| IBIS file stm32u575_585_lqfp64.ibs
[IBIS ver] 4.2
[File name] stm32u575_585_lqfp64.ibs
[File Rev] 1.0
[Date]   06-08-2021
[Source] Data Created at STMicroelectronics
[Notes]  File originated from ELDO simulations.
[Disclaimer]  This information is for modeling purpose only and is
   not guaranted. The information is subject to change without
   notice.
[Copyright] Copyright 2021 STMicroelectronics Inc.
|   Component stm32u575_585_lqfp64
[Component] stm32u575_585_lqfp64
[Manufacturer] STMicroelectronics
[Package]
| variable   typ   min   max
R_pkg   0   NA   NA
L_pkg   0   NA   NA
C_pkg   0   NA   NA
[Pin]   signal_name   model_name   R_pin   L_pin   C_pin   | Comment
1 VBAT POWER 68.980E-3 4.220E-9 120.000E-15
2 PC13 io8_100m_ft_v33 63.756E-3 3.679E-9 93.469E-15
3 PC14-OSC32_IN io8_100m_ft 59.336E-3 3.221E-9 71.020E-15
4 PC15-OSC32_OUT io8_100m_ft 55.719E-3 2.846E-9 52.653E-15
5 PH0-OSC_IN io8_100m_ft 52.907E-3 2.555E-9 38.367E-15
6 PH1-OSC_OUT io8_100m_ft 50.897E-3 2.347E-9 28.163E-15
7 NRST nc 49.692E-3 2.222E-9 22.041E-15
8 PC0 io8_100m_hslv_ft 49.290E-3 2.180E-9 20.000E-15
9 PC1 io8_166m_hslv_i2c_ft 49.290E-3 2.180E-9 20.000E-15
10 PC2 io8_100m_hslv_ft 49.692E-3 2.222E-9 22.041E-15
11 PC3 io8_100m_hslv_ft 50.897E-3 2.347E-9 28.163E-15
12 VSSA GND 52.907E-3 2.555E-9 38.367E-15
13 VDDA POWER 55.719E-3 2.846E-9 52.653E-15
14 PA0 io8_100m_hslv_tamp_ft 59.336E-3 3.221E-9 71.020E-15
15 PA1 io8_100m_hslv_tamp_ft 63.756E-3 3.679E-9 93.469E-15
16 PA2 io8_100m_hslv_ft 68.980E-3 4.220E-9 120.000E-15
17 PA3 io8_166m_hslv_ft 68.980E-3 4.220E-9 120.000E-15
18 VSS GND 63.756E-3 3.679E-9 93.469E-15
19 VDD POWER 59.336E-3 3.221E-9 71.020E-15
20 PA4 io8_100m_hslv_ft 55.719E-3 2.846E-9 52.653E-15
21 PA5 io8_100m_ft 52.907E-3 2.555E-9 38.367E-15
22 PA6 io8_100m_hslv_ft 50.897E-3 2.347E-9 28.163E-15
23 PA7 io8_100m_hslv_ft 49.692E-3 2.222E-9 22.041E-15
24 PC4 io8_100m_hslv_ft 49.290E-3 2.180E-9 20.000E-15
25 PC5 io8_100m_tamp_ft 49.290E-3 2.180E-9 20.000E-15
26 PB0 io8_100m_hslv_ft 49.692E-3 2.222E-9 22.041E-15
27 PB1 io8_100m_hslv_ft 50.897E-3 2.347E-9 28.163E-15
28 PB2 io8_100m_hslv_tamp_ft 52.907E-3 2.555E-9 38.367E-15
29 PB10 io8_166m_hslv_i2c_ft 55.719E-3 2.846E-9 52.653E-15
30 VCAP POWER 59.336E-3 3.221E-9 71.020E-15
31 VSS GND 63.756E-3 3.679E-9 93.469E-15
32 VDD POWER 68.980E-3 4.220E-9 120.000E-15
33 PB12 io8_166m_hslv_ft 68.980E-3 4.220E-9 120.000E-15
34 PB13 io8_100m_i2c_ft 63.756E-3 3.679E-9 93.469E-15
35 PB14 io8_100m_i2c_ft 59.336E-3 3.221E-9 71.020E-15
36 PB15 nc 55.719E-3 2.846E-9 52.653E-15
37 PC6 io8_100m_ft 52.907E-3 2.555E-9 38.367E-15
38 PC7 io8_100m_ft 50.897E-3 2.347E-9 28.163E-15
39 PC8 io8_100m_ft 49.692E-3 2.222E-9 22.041E-15
40 PC9 io8_100m_ft 49.290E-3 2.180E-9 20.000E-15
41 PA8 io8_166m_hslv_ft 49.290E-3 2.180E-9 20.000E-15
42 PA9 io8_100m_usb_vbus_ft 49.692E-3 2.222E-9 22.041E-15
43 PA10 io8_100m_usb_id 50.897E-3 2.347E-9 28.163E-15
44 PA11 io8_usb_ft 52.907E-3 2.555E-9 38.367E-15
45 PA12 io8_usb_ft 55.719E-3 2.846E-9 52.653E-15
46 PA13 io8_100m_ft 59.336E-3 3.221E-9 71.020E-15
47 VSSUSB GND 63.756E-3 3.679E-9 93.469E-15
48 VDDUSB POWER 68.980E-3 4.220E-9 120.000E-15
49 PA14 io8_100m_ft 68.980E-3 4.220E-9 120.000E-15
50 PA15 nc 63.756E-3 3.679E-9 93.469E-15
51 PC10 io8_100m_ft 59.336E-3 3.221E-9 71.020E-15
52 PC11 io8_100m_hslv_ft 55.719E-3 2.846E-9 52.653E-15
53 PC12 io8_166m_hslv_ft 52.907E-3 2.555E-9 38.367E-15
54 PD2 io8_100m_ft 50.897E-3 2.347E-9 28.163E-15
55 PB3 io8_100m_i2c_ft 49.692E-3 2.222E-9 22.041E-15
56 PB4 io8_100m_i2c_ft 49.290E-3 2.180E-9 20.000E-15
57 PB5 io8_166m_hslv_ft 49.290E-3 2.180E-9 20.000E-15
58 PB6 io8_100m_i2c_ft 49.692E-3 2.222E-9 22.041E-15
59 PB7 io8_166m_hslv_i2c_ft 50.897E-3 2.347E-9 28.163E-15
60 PH3-BOOT0 io8_100m_ft 52.907E-3 2.555E-9 38.367E-15
61 PB8 io8_100m_i2c_ft 55.719E-3 2.846E-9 52.653E-15
62 PB9 io8_100m_i2c_ft 59.336E-3 3.221E-9 71.020E-15
63 VSS GND 63.756E-3 3.679E-9 93.469E-15
64 VDD POWER 68.980E-3 4.220E-9 120.000E-15
[Model Selector] io8_100m_ft
io8_100m_ft_hs_1v2  "IO8_FT 100MHz high speed @ 1.2V"
io8_100m_ft_hs_pu_1v2  "IO8_FT 100MHz high speed @ 1.2V pullup"
io8_100m_ft_hs_pd_1v2  "IO8_FT 100MHz high speed @ 1.2V pulldown"
io8_100m_ft_fs_1v2  "IO8_FT 100MHz fast speed @ 1.2V"
io8_100m_ft_fs_pu_1v2  "IO8_FT 100MHz fast speed @ 1.2V pullup"
io8_100m_ft_fs_pd_1v2  "IO8_FT 100MHz fast speed @ 1.2V pulldown"
io8_100m_ft_ms_1v2  "IO8_FT 100MHz med speed @ 1.2V"
io8_100m_ft_ms_pu_1v2  "IO8_FT 100MHz med speed @ 1.2V pullup"
io8_100m_ft_ms_pd_1v2  "IO8_FT 100MHz med speed @ 1.2V pulldown"
io8_100m_ft_ls_1v2  "IO8_FT 100MHz low speed @ 1.2V"
io8_100m_ft_ls_pu_1v2  "IO8_FT 100MHz low speed @ 1.2V pullup"
io8_100m_ft_ls_pd_1v2  "IO8_FT 100MHz low speed @ 1.2V pulldown"
io8_100m_ft_hs_1v8  "IO8_FT 100MHz high speed @ 1.8V"
io8_100m_ft_hs_pu_1v8  "IO8_FT 100MHz high speed @ 1.8V pullup"
io8_100m_ft_hs_pd_1v8  "IO8_FT 100MHz high speed @ 1.8V pulldown"
io8_100m_ft_fs_1v8  "IO8_FT 100MHz fast speed @ 1.8V"
io8_100m_ft_fs_pu_1v8  "IO8_FT 100MHz fast speed @ 1.8V pullup"
io8_100m_ft_fs_pd_1v8  "IO8_FT 100MHz fast speed @ 1.8V pulldown"
io8_100m_ft_ms_1v8  "IO8_FT 100MHz med speed @ 1.8V"
io8_100m_ft_ms_pu_1v8  "IO8_FT 100MHz med speed @ 1.8V pullup"
io8_100m_ft_ms_pd_1v8  "IO8_FT 100MHz med speed @ 1.8V pulldown"
io8_100m_ft_ls_1v8  "IO8_FT 100MHz low speed @ 1.8V"
io8_100m_ft_ls_pu_1v8  "IO8_FT 100MHz low speed @ 1.8V pullup"
io8_100m_ft_ls_pd_1v8  "IO8_FT 100MHz low speed @ 1.8V pulldown"
io8_100m_ft_hs_3v3  "IO8_FT 100MHz high speed @ 3.3V"
io8_100m_ft_hs_pu_3v3  "IO8_FT 100MHz high speed @ 3.3V pullup"
io8_100m_ft_hs_pd_3v3  "IO8_FT 100MHz high speed @ 3.3V pulldown"
io8_100m_ft_fs_3v3  "IO8_FT 100MHz fast speed @ 3.3V"
io8_100m_ft_fs_pu_3v3  "IO8_FT 100MHz fast speed @ 3.3V pullup"
io8_100m_ft_fs_pd_3v3  "IO8_FT 100MHz fast speed @ 3.3V pulldown"
io8_100m_ft_ms_3v3  "IO8_FT 100MHz med speed @ 3.3V"
io8_100m_ft_ms_pu_3v3  "IO8_FT 100MHz med speed @ 3.3V pullup"
io8_100m_ft_ms_pd_3v3  "IO8_FT 100MHz med speed @ 3.3V pulldown"
io8_100m_ft_ls_3v3  "IO8_FT 100MHz low speed @ 3.3V"
io8_100m_ft_ls_pu_3v3  "IO8_FT 100MHz low speed @ 3.3V pullup"
io8_100m_ft_ls_pd_3v3  "IO8_FT 100MHz low speed @ 3.3V pulldown"
[Model Selector] io8_100m_hslv_ft
io8_100m_ft_hs_1v2  "IO8_FT 100MHz high speed @ 1.2V"
io8_100m_ft_hs_pu_1v2  "IO8_FT 100MHz high speed @ 1.2V pullup"
io8_100m_ft_hs_pd_1v2  "IO8_FT 100MHz high speed @ 1.2V pulldown"
io8_100m_ft_fs_1v2  "IO8_FT 100MHz fast speed @ 1.2V"
io8_100m_ft_fs_pu_1v2  "IO8_FT 100MHz fast speed @ 1.2V pullup"
io8_100m_ft_fs_pd_1v2  "IO8_FT 100MHz fast speed @ 1.2V pulldown"
io8_100m_ft_ms_1v2  "IO8_FT 100MHz med speed @ 1.2V"
io8_100m_ft_ms_pu_1v2  "IO8_FT 100MHz med speed @ 1.2V pullup"
io8_100m_ft_ms_pd_1v2  "IO8_FT 100MHz med speed @ 1.2V pulldown"
io8_100m_ft_ls_1v2  "IO8_FT 100MHz low speed @ 1.2V"
io8_100m_ft_ls_pu_1v2  "IO8_FT 100MHz low speed @ 1.2V pullup"
io8_100m_ft_ls_pd_1v2  "IO8_FT 100MHz low speed @ 1.2V pulldown"
io8_100m_ft_hs_1v8  "IO8_FT 100MHz high speed @ 1.8V"
io8_100m_ft_hs_pu_1v8  "IO8_FT 100MHz high speed @ 1.8V pullup"
io8_100m_ft_hs_pd_1v8  "IO8_FT 100MHz high speed @ 1.8V pulldown"
io8_100m_ft_fs_1v8  "IO8_FT 100MHz fast speed @ 1.8V"
io8_100m_ft_fs_pu_1v8  "IO8_FT 100MHz fast speed @ 1.8V pullup"
io8_100m_ft_fs_pd_1v8  "IO8_FT 100MHz fast speed @ 1.8V pulldown"
io8_100m_ft_ms_1v8  "IO8_FT 100MHz med speed @ 1.8V"
io8_100m_ft_ms_pu_1v8  "IO8_FT 100MHz med speed @ 1.8V pullup"
io8_100m_ft_ms_pd_1v8  "IO8_FT 100MHz med speed @ 1.8V pulldown"
io8_100m_ft_ls_1v8  "IO8_FT 100MHz low speed @ 1.8V"
io8_100m_ft_ls_pu_1v8  "IO8_FT 100MHz low speed @ 1.8V pullup"
io8_100m_ft_ls_pd_1v8  "IO8_FT 100MHz low speed @ 1.8V pulldown"
io8_100m_ft_hs_3v3  "IO8_FT 100MHz high speed @ 3.3V"
io8_100m_ft_hs_pu_3v3  "IO8_FT 100MHz high speed @ 3.3V pullup"
io8_100m_ft_hs_pd_3v3  "IO8_FT 100MHz high speed @ 3.3V pulldown"
io8_100m_ft_fs_3v3  "IO8_FT 100MHz fast speed @ 3.3V"
io8_100m_ft_fs_pu_3v3  "IO8_FT 100MHz fast speed @ 3.3V pullup"
io8_100m_ft_fs_pd_3v3  "IO8_FT 100MHz fast speed @ 3.3V pulldown"
io8_100m_ft_ms_3v3  "IO8_FT 100MHz med speed @ 3.3V"
io8_100m_ft_ms_pu_3v3  "IO8_FT 100MHz med speed @ 3.3V pullup"
io8_100m_ft_ms_pd_3v3  "IO8_FT 100MHz med speed @ 3.3V pulldown"
io8_100m_ft_ls_3v3  "IO8_FT 100MHz low speed @ 3.3V"
io8_100m_ft_ls_pu_3v3  "IO8_FT 100MHz low speed @ 3.3V pullup"
io8_100m_ft_ls_pd_3v3  "IO8_FT 100MHz low speed @ 3.3V pulldown"
io8_100m_hslv_ft_hs_1v2  "IO8_FT 100MHz HSLV high speed @ 1.2V"
io8_100m_hslv_ft_hs_pu_1v2  "IO8_FT 100MHz HSLV high speed @ 1.2V pullup"
io8_100m_hslv_ft_hs_pd_1v2  "IO8_FT 100MHz HSLV high speed @ 1.2V pulldown"
io8_100m_hslv_ft_fs_1v2  "IO8_FT 100MHz HSLV fast speed @ 1.2V"
io8_100m_hslv_ft_fs_pu_1v2  "IO8_FT 100MHz HSLV fast speed @ 1.2V pullup"
io8_100m_hslv_ft_fs_pd_1v2  "IO8_FT 100MHz HSLV fast speed @ 1.2V pulldown"
io8_100m_hslv_ft_ms_1v2  "IO8_FT 100MHz HSLV med speed @ 1.2V"
io8_100m_hslv_ft_ms_pu_1v2  "IO8_FT 100MHz HSLV med speed @ 1.2V pullup"
io8_100m_hslv_ft_ms_pd_1v2  "IO8_FT 100MHz HSLV med speed @ 1.2V pulldown"
io8_100m_hslv_ft_ls_1v2  "IO8_FT 100MHz HSLV low speed @ 1.2V"
io8_100m_hslv_ft_ls_pu_1v2  "IO8_FT 100MHz HSLV low speed @ 1.2V pullup"
io8_100m_hslv_ft_ls_pd_1v2  "IO8_FT 100MHz HSLV low speed @ 1.2V pulldown"
io8_100m_hslv_ft_hs_1v8  "IO8_FT 100MHz HSLV high speed @ 1.8V"
io8_100m_hslv_ft_hs_pu_1v8  "IO8_FT 100MHz HSLV high speed @ 1.8V pullup"
io8_100m_hslv_ft_hs_pd_1v8  "IO8_FT 100MHz HSLV high speed @ 1.8V pulldown"
io8_100m_hslv_ft_fs_1v8  "IO8_FT 100MHz HSLV fast speed @ 1.8V"
io8_100m_hslv_ft_fs_pu_1v8  "IO8_FT 100MHz HSLV fast speed @ 1.8V pullup"
io8_100m_hslv_ft_fs_pd_1v8  "IO8_FT 100MHz HSLV fast speed @ 1.8V pulldown"
io8_100m_hslv_ft_ms_1v8  "IO8_FT 100MHz HSLV med speed @ 1.8V"
io8_100m_hslv_ft_ms_pu_1v8  "IO8_FT 100MHz HSLV med speed @ 1.8V pullup"
io8_100m_hslv_ft_ms_pd_1v8  "IO8_FT 100MHz HSLV med speed @ 1.8V pulldown"
io8_100m_hslv_ft_ls_1v8  "IO8_FT 100MHz HSLV low speed @ 1.8V"
io8_100m_hslv_ft_ls_pu_1v8  "IO8_FT 100MHz HSLV low speed @ 1.8V pullup"
io8_100m_hslv_ft_ls_pd_1v8  "IO8_FT 100MHz HSLV low speed @ 1.8V pulldown"
io8_100m_hslv_ft_hs_2v5  "IO8_FT 100MHz HSLV high speed @ 2.5V"
io8_100m_hslv_ft_hs_pu_2v5  "IO8_FT 100MHz HSLV high speed @ 2.5V pullup"
io8_100m_hslv_ft_hs_pd_2v5  "IO8_FT 100MHz HSLV high speed @ 2.5V pulldown"
io8_100m_hslv_ft_fs_2v5  "IO8_FT 100MHz HSLV fast speed @ 2.5V"
io8_100m_hslv_ft_fs_pu_2v5  "IO8_FT 100MHz HSLV fast speed @ 2.5V pullup"
io8_100m_hslv_ft_fs_pd_2v5  "IO8_FT 100MHz HSLV fast speed @ 2.5V pulldown"
io8_100m_hslv_ft_ms_2v5  "IO8_FT 100MHz HSLV med speed @ 2.5V"
io8_100m_hslv_ft_ms_pu_2v5  "IO8_FT 100MHz HSLV med speed @ 2.5V pullup"
io8_100m_hslv_ft_ms_pd_2v5  "IO8_FT 100MHz HSLV med speed @ 2.5V pulldown"
io8_100m_hslv_ft_ls_2v5  "IO8_FT 100MHz HSLV low speed @ 2.5V"
io8_100m_hslv_ft_ls_pu_2v5  "IO8_FT 100MHz HSLV low speed @ 2.5V pullup"
io8_100m_hslv_ft_ls_pd_2v5  "IO8_FT 100MHz HSLV low speed @ 2.5V pulldown"
[Model Selector] io8_166m_hslv_ft
io8_166m_ft_hs_1v2  "IO8_FT 166MHz high speed @ 1.2V"
io8_166m_ft_hs_pu_1v2  "IO8_FT 166MHz high speed @ 1.2V pullup"
io8_166m_ft_hs_pd_1v2  "IO8_FT 166MHz high speed @ 1.2V pulldown"
io8_166m_ft_fs_1v2  "IO8_FT 166MHz fast speed @ 1.2V"
io8_166m_ft_fs_pu_1v2  "IO8_FT 166MHz fast speed @ 1.2V pullup"
io8_166m_ft_fs_pd_1v2  "IO8_FT 166MHz fast speed @ 1.2V pulldown"
io8_166m_ft_ms_1v2  "IO8_FT 166MHz med speed @ 1.2V"
io8_166m_ft_ms_pu_1v2  "IO8_FT 166MHz med speed @ 1.2V pullup"
io8_166m_ft_ms_pd_1v2  "IO8_FT 166MHz med speed @ 1.2V pulldown"
io8_166m_ft_ls_1v2  "IO8_FT 166MHz low speed @ 1.2V"
io8_166m_ft_ls_pu_1v2  "IO8_FT 166MHz low speed @ 1.2V pullup"
io8_166m_ft_ls_pd_1v2  "IO8_FT 166MHz low speed @ 1.2V pulldown"
io8_166m_ft_hs_1v8  "IO8_FT 166MHz high speed @ 1.8V"
io8_166m_ft_hs_pu_1v8  "IO8_FT 166MHz high speed @ 1.8V pullup"
io8_166m_ft_hs_pd_1v8  "IO8_FT 166MHz high speed @ 1.8V pulldown"
io8_166m_ft_fs_1v8  "IO8_FT 166MHz fast speed @ 1.8V"
io8_166m_ft_fs_pu_1v8  "IO8_FT 166MHz fast speed @ 1.8V pullup"
io8_166m_ft_fs_pd_1v8  "IO8_FT 166MHz fast speed @ 1.8V pulldown"
io8_166m_ft_ms_1v8  "IO8_FT 166MHz med speed @ 1.8V"
io8_166m_ft_ms_pu_1v8  "IO8_FT 166MHz med speed @ 1.8V pullup"
io8_166m_ft_ms_pd_1v8  "IO8_FT 166MHz med speed @ 1.8V pulldown"
io8_166m_ft_ls_1v8  "IO8_FT 166MHz low speed @ 1.8V"
io8_166m_ft_ls_pu_1v8  "IO8_FT 166MHz low speed @ 1.8V pullup"
io8_166m_ft_ls_pd_1v8  "IO8_FT 166MHz low speed @ 1.8V pulldown"
io8_166m_ft_hs_3v3  "IO8_FT 166MHz high speed @ 3.3V"
io8_166m_ft_hs_pu_3v3  "IO8_FT 166MHz high speed @ 3.3V pullup"
io8_166m_ft_hs_pd_3v3  "IO8_FT 166MHz high speed @ 3.3V pulldown"
io8_166m_ft_fs_3v3  "IO8_FT 166MHz fast speed @ 3.3V"
io8_166m_ft_fs_pu_3v3  "IO8_FT 166MHz fast speed @ 3.3V pullup"
io8_166m_ft_fs_pd_3v3  "IO8_FT 166MHz fast speed @ 3.3V pulldown"
io8_166m_ft_ms_3v3  "IO8_FT 166MHz med speed @ 3.3V"
io8_166m_ft_ms_pu_3v3  "IO8_FT 166MHz med speed @ 3.3V pullup"
io8_166m_ft_ms_pd_3v3  "IO8_FT 166MHz med speed @ 3.3V pulldown"
io8_166m_ft_ls_3v3  "IO8_FT 166MHz low speed @ 3.3V"
io8_166m_ft_ls_pu_3v3  "IO8_FT 166MHz low speed @ 3.3V pullup"
io8_166m_ft_ls_pd_3v3  "IO8_FT 166MHz low speed @ 3.3V pulldown"
io8_166m_hslv_ft_hs_1v2  "IO8_FT 166MHz HSLV high speed @ 1.2V"
io8_166m_hslv_ft_hs_pu_1v2  "IO8_FT 166MHz HSLV high speed @ 1.2V pullup"
io8_166m_hslv_ft_hs_pd_1v2  "IO8_FT 166MHz HSLV high speed @ 1.2V pulldown"
io8_166m_hslv_ft_fs_1v2  "IO8_FT 166MHz HSLV fast speed @ 1.2V"
io8_166m_hslv_ft_fs_pu_1v2  "IO8_FT 166MHz HSLV fast speed @ 1.2V pullup"
io8_166m_hslv_ft_fs_pd_1v2  "IO8_FT 166MHz HSLV fast speed @ 1.2V pulldown"
io8_166m_hslv_ft_ms_1v2  "IO8_FT 166MHz HSLV med speed @ 1.2V"
io8_166m_hslv_ft_ms_pu_1v2  "IO8_FT 166MHz HSLV med speed @ 1.2V pullup"
io8_166m_hslv_ft_ms_pd_1v2  "IO8_FT 166MHz HSLV med speed @ 1.2V pulldown"
io8_166m_hslv_ft_ls_1v2  "IO8_FT 166MHz HSLV low speed @ 1.2V"
io8_166m_hslv_ft_ls_pu_1v2  "IO8_FT 166MHz HSLV low speed @ 1.2V pullup"
io8_166m_hslv_ft_ls_pd_1v2  "IO8_FT 166MHz HSLV low speed @ 1.2V pulldown"
io8_166m_hslv_ft_hs_1v8  "IO8_FT 166MHz HSLV high speed @ 1.8V"
io8_166m_hslv_ft_hs_pu_1v8  "IO8_FT 166MHz HSLV high speed @ 1.8V pullup"
io8_166m_hslv_ft_hs_pd_1v8  "IO8_FT 166MHz HSLV high speed @ 1.8V pulldown"
io8_166m_hslv_ft_fs_1v8  "IO8_FT 166MHz HSLV fast speed @ 1.8V"
io8_166m_hslv_ft_fs_pu_1v8  "IO8_FT 166MHz HSLV fast speed @ 1.8V pullup"
io8_166m_hslv_ft_fs_pd_1v8  "IO8_FT 166MHz HSLV fast speed @ 1.8V pulldown"
io8_166m_hslv_ft_ms_1v8  "IO8_FT 166MHz HSLV med speed @ 1.8V"
io8_166m_hslv_ft_ms_pu_1v8  "IO8_FT 166MHz HSLV med speed @ 1.8V pullup"
io8_166m_hslv_ft_ms_pd_1v8  "IO8_FT 166MHz HSLV med speed @ 1.8V pulldown"
io8_166m_hslv_ft_ls_1v8  "IO8_FT 166MHz HSLV low speed @ 1.8V"
io8_166m_hslv_ft_ls_pu_1v8  "IO8_FT 166MHz HSLV low speed @ 1.8V pullup"
io8_166m_hslv_ft_ls_pd_1v8  "IO8_FT 166MHz HSLV low speed @ 1.8V pulldown"
io8_166m_hslv_ft_hs_2v5  "IO8_FT 166MHz HSLV high speed @ 2.5V"
io8_166m_hslv_ft_hs_pu_2v5  "IO8_FT 166MHz HSLV high speed @ 2.5V pullup"
io8_166m_hslv_ft_hs_pd_2v5  "IO8_FT 166MHz HSLV high speed @ 2.5V pulldown"
io8_166m_hslv_ft_fs_2v5  "IO8_FT 166MHz HSLV fast speed @ 2.5V"
io8_166m_hslv_ft_fs_pu_2v5  "IO8_FT 166MHz HSLV fast speed @ 2.5V pullup"
io8_166m_hslv_ft_fs_pd_2v5  "IO8_FT 166MHz HSLV fast speed @ 2.5V pulldown"
io8_166m_hslv_ft_ms_2v5  "IO8_FT 166MHz HSLV med speed @ 2.5V"
io8_166m_hslv_ft_ms_pu_2v5  "IO8_FT 166MHz HSLV med speed @ 2.5V pullup"
io8_166m_hslv_ft_ms_pd_2v5  "IO8_FT 166MHz HSLV med speed @ 2.5V pulldown"
io8_166m_hslv_ft_ls_2v5  "IO8_FT 166MHz HSLV low speed @ 2.5V"
io8_166m_hslv_ft_ls_pu_2v5  "IO8_FT 166MHz HSLV low speed @ 2.5V pullup"
io8_166m_hslv_ft_ls_pd_2v5  "IO8_FT 166MHz HSLV low speed @ 2.5V pulldown"
[Model Selector] io8_100m_ft_v33
io8_ft_v33_hs_1v2  "IO8_FT_V33 high speed @ 1.2V"
io8_ft_v33_hs_pu_1v2  "IO8_FT_V33 high speed @ 1.2V pullup"
io8_ft_v33_hs_pd_1v2  "IO8_FT_V33 high speed @ 1.2V pulldown"
io8_ft_v33_fs_1v2  "IO8_FT_V33 fast speed @ 1.2V"
io8_ft_v33_fs_pu_1v2  "IO8_FT_V33 fast speed @ 1.2V pullup"
io8_ft_v33_fs_pd_1v2  "IO8_FT_V33 fast speed @ 1.2V pulldown"
io8_ft_v33_ms_1v2  "IO8_FT_V33 med speed @ 1.2V"
io8_ft_v33_ms_pu_1v2  "IO8_FT_V33 med speed @ 1.2V pullup"
io8_ft_v33_ms_pd_1v2  "IO8_FT_V33 med speed @ 1.2V pulldown"
io8_ft_v33_ls_1v2  "IO8_FT_V33 low speed @ 1.2V"
io8_ft_v33_ls_pu_1v2  "IO8_FT_V33 low speed @ 1.2V pullup"
io8_ft_v33_ls_pd_1v2  "IO8_FT_V33 low speed @ 1.2V pulldown"
io8_ft_v33_hs_1v8  "IO8_FT_V33 high speed @ 1.8V"
io8_ft_v33_hs_pu_1v8  "IO8_FT_V33 high speed @ 1.8V pullup"
io8_ft_v33_hs_pd_1v8  "IO8_FT_V33 high speed @ 1.8V pulldown"
io8_ft_v33_fs_1v8  "IO8_FT_V33 fast speed @ 1.8V"
io8_ft_v33_fs_pu_1v8  "IO8_FT_V33 fast speed @ 1.8V pullup"
io8_ft_v33_fs_pd_1v8  "IO8_FT_V33 fast speed @ 1.8V pulldown"
io8_ft_v33_ms_1v8  "IO8_FT_V33 med speed @ 1.8V"
io8_ft_v33_ms_pu_1v8  "IO8_FT_V33 med speed @ 1.8V pullup"
io8_ft_v33_ms_pd_1v8  "IO8_FT_V33 med speed @ 1.8V pulldown"
io8_ft_v33_ls_1v8  "IO8_FT_V33 low speed @ 1.8V"
io8_ft_v33_ls_pu_1v8  "IO8_FT_V33 low speed @ 1.8V pullup"
io8_ft_v33_ls_pd_1v8  "IO8_FT_V33 low speed @ 1.8V pulldown"
io8_ft_v33_hs_3v3  "IO8_FT_V33 high speed @ 3.3V"
io8_ft_v33_hs_pu_3v3  "IO8_FT_V33 high speed @ 3.3V pullup"
io8_ft_v33_hs_pd_3v3  "IO8_FT_V33 high speed @ 3.3V pulldown"
io8_ft_v33_fs_3v3  "IO8_FT_V33 fast speed @ 3.3V"
io8_ft_v33_fs_pu_3v3  "IO8_FT_V33 fast speed @ 3.3V pullup"
io8_ft_v33_fs_pd_3v3  "IO8_FT_V33 fast speed @ 3.3V pulldown"
io8_ft_v33_ms_3v3  "IO8_FT_V33 med speed @ 3.3V"
io8_ft_v33_ms_pu_3v3  "IO8_FT_V33 med speed @ 3.3V pullup"
io8_ft_v33_ms_pd_3v3  "IO8_FT_V33 med speed @ 3.3V pulldown"
io8_ft_v33_ls_3v3  "IO8_FT_V33 low speed @ 3.3V"
io8_ft_v33_ls_pu_3v3  "IO8_FT_V33 low speed @ 3.3V pullup"
io8_ft_v33_ls_pd_3v3  "IO8_FT_V33 low speed @ 3.3V pulldown"
[Model Selector] io8_100m_tamp_ft
io8_100m_ft_hs_1v2  "IO8_FT 100MHz high speed @ 1.2V"
io8_100m_ft_hs_pu_1v2  "IO8_FT 100MHz high speed @ 1.2V pullup"
io8_100m_ft_hs_pd_1v2  "IO8_FT 100MHz high speed @ 1.2V pulldown"
io8_100m_ft_fs_1v2  "IO8_FT 100MHz fast speed @ 1.2V"
io8_100m_ft_fs_pu_1v2  "IO8_FT 100MHz fast speed @ 1.2V pullup"
io8_100m_ft_fs_pd_1v2  "IO8_FT 100MHz fast speed @ 1.2V pulldown"
io8_100m_ft_ms_1v2  "IO8_FT 100MHz med speed @ 1.2V"
io8_100m_ft_ms_pu_1v2  "IO8_FT 100MHz med speed @ 1.2V pullup"
io8_100m_ft_ms_pd_1v2  "IO8_FT 100MHz med speed @ 1.2V pulldown"
io8_100m_ft_ls_1v2  "IO8_FT 100MHz low speed @ 1.2V"
io8_100m_ft_ls_pu_1v2  "IO8_FT 100MHz low speed @ 1.2V pullup"
io8_100m_ft_ls_pd_1v2  "IO8_FT 100MHz low speed @ 1.2V pulldown"
io8_100m_ft_hs_1v8  "IO8_FT 100MHz high speed @ 1.8V"
io8_100m_ft_hs_pu_1v8  "IO8_FT 100MHz high speed @ 1.8V pullup"
io8_100m_ft_hs_pd_1v8  "IO8_FT 100MHz high speed @ 1.8V pulldown"
io8_100m_ft_fs_1v8  "IO8_FT 100MHz fast speed @ 1.8V"
io8_100m_ft_fs_pu_1v8  "IO8_FT 100MHz fast speed @ 1.8V pullup"
io8_100m_ft_fs_pd_1v8  "IO8_FT 100MHz fast speed @ 1.8V pulldown"
io8_100m_ft_ms_1v8  "IO8_FT 100MHz med speed @ 1.8V"
io8_100m_ft_ms_pu_1v8  "IO8_FT 100MHz med speed @ 1.8V pullup"
io8_100m_ft_ms_pd_1v8  "IO8_FT 100MHz med speed @ 1.8V pulldown"
io8_100m_ft_ls_1v8  "IO8_FT 100MHz low speed @ 1.8V"
io8_100m_ft_ls_pu_1v8  "IO8_FT 100MHz low speed @ 1.8V pullup"
io8_100m_ft_ls_pd_1v8  "IO8_FT 100MHz low speed @ 1.8V pulldown"
io8_100m_ft_hs_3v3  "IO8_FT 100MHz high speed @ 3.3V"
io8_100m_ft_hs_pu_3v3  "IO8_FT 100MHz high speed @ 3.3V pullup"
io8_100m_ft_hs_pd_3v3  "IO8_FT 100MHz high speed @ 3.3V pulldown"
io8_100m_ft_fs_3v3  "IO8_FT 100MHz fast speed @ 3.3V"
io8_100m_ft_fs_pu_3v3  "IO8_FT 100MHz fast speed @ 3.3V pullup"
io8_100m_ft_fs_pd_3v3  "IO8_FT 100MHz fast speed @ 3.3V pulldown"
io8_100m_ft_ms_3v3  "IO8_FT 100MHz med speed @ 3.3V"
io8_100m_ft_ms_pu_3v3  "IO8_FT 100MHz med speed @ 3.3V pullup"
io8_100m_ft_ms_pd_3v3  "IO8_FT 100MHz med speed @ 3.3V pulldown"
io8_100m_ft_ls_3v3  "IO8_FT 100MHz low speed @ 3.3V"
io8_100m_ft_ls_pu_3v3  "IO8_FT 100MHz low speed @ 3.3V pullup"
io8_100m_ft_ls_pd_3v3  "IO8_FT 100MHz low speed @ 3.3V pulldown"
io8_ft_v33_hs_1v2  "IO8_FT_V33 high speed @ 1.2V"
io8_ft_v33_hs_pu_1v2  "IO8_FT_V33 high speed @ 1.2V pullup"
io8_ft_v33_hs_pd_1v2  "IO8_FT_V33 high speed @ 1.2V pulldown"
io8_ft_v33_fs_1v2  "IO8_FT_V33 fast speed @ 1.2V"
io8_ft_v33_fs_pu_1v2  "IO8_FT_V33 fast speed @ 1.2V pullup"
io8_ft_v33_fs_pd_1v2  "IO8_FT_V33 fast speed @ 1.2V pulldown"
io8_ft_v33_ms_1v2  "IO8_FT_V33 med speed @ 1.2V"
io8_ft_v33_ms_pu_1v2  "IO8_FT_V33 med speed @ 1.2V pullup"
io8_ft_v33_ms_pd_1v2  "IO8_FT_V33 med speed @ 1.2V pulldown"
io8_ft_v33_ls_1v2  "IO8_FT_V33 low speed @ 1.2V"
io8_ft_v33_ls_pu_1v2  "IO8_FT_V33 low speed @ 1.2V pullup"
io8_ft_v33_ls_pd_1v2  "IO8_FT_V33 low speed @ 1.2V pulldown"
io8_ft_v33_hs_1v8  "IO8_FT_V33 high speed @ 1.8V"
io8_ft_v33_hs_pu_1v8  "IO8_FT_V33 high speed @ 1.8V pullup"
io8_ft_v33_hs_pd_1v8  "IO8_FT_V33 high speed @ 1.8V pulldown"
io8_ft_v33_fs_1v8  "IO8_FT_V33 fast speed @ 1.8V"
io8_ft_v33_fs_pu_1v8  "IO8_FT_V33 fast speed @ 1.8V pullup"
io8_ft_v33_fs_pd_1v8  "IO8_FT_V33 fast speed @ 1.8V pulldown"
io8_ft_v33_ms_1v8  "IO8_FT_V33 med speed @ 1.8V"
io8_ft_v33_ms_pu_1v8  "IO8_FT_V33 med speed @ 1.8V pullup"
io8_ft_v33_ms_pd_1v8  "IO8_FT_V33 med speed @ 1.8V pulldown"
io8_ft_v33_ls_1v8  "IO8_FT_V33 low speed @ 1.8V"
io8_ft_v33_ls_pu_1v8  "IO8_FT_V33 low speed @ 1.8V pullup"
io8_ft_v33_ls_pd_1v8  "IO8_FT_V33 low speed @ 1.8V pulldown"
io8_ft_v33_hs_3v3  "IO8_FT_V33 high speed @ 3.3V"
io8_ft_v33_hs_pu_3v3  "IO8_FT_V33 high speed @ 3.3V pullup"
io8_ft_v33_hs_pd_3v3  "IO8_FT_V33 high speed @ 3.3V pulldown"
io8_ft_v33_fs_3v3  "IO8_FT_V33 fast speed @ 3.3V"
io8_ft_v33_fs_pu_3v3  "IO8_FT_V33 fast speed @ 3.3V pullup"
io8_ft_v33_fs_pd_3v3  "IO8_FT_V33 fast speed @ 3.3V pulldown"
io8_ft_v33_ms_3v3  "IO8_FT_V33 med speed @ 3.3V"
io8_ft_v33_ms_pu_3v3  "IO8_FT_V33 med speed @ 3.3V pullup"
io8_ft_v33_ms_pd_3v3  "IO8_FT_V33 med speed @ 3.3V pulldown"
io8_ft_v33_ls_3v3  "IO8_FT_V33 low speed @ 3.3V"
io8_ft_v33_ls_pu_3v3  "IO8_FT_V33 low speed @ 3.3V pullup"
io8_ft_v33_ls_pd_3v3  "IO8_FT_V33 low speed @ 3.3V pulldown"
[Model Selector] io8_100m_hslv_tamp_ft
io8_100m_ft_hs_1v2  "IO8_FT 100MHz high speed @ 1.2V"
io8_100m_ft_hs_pu_1v2  "IO8_FT 100MHz high speed @ 1.2V pullup"
io8_100m_ft_hs_pd_1v2  "IO8_FT 100MHz high speed @ 1.2V pulldown"
io8_100m_ft_fs_1v2  "IO8_FT 100MHz fast speed @ 1.2V"
io8_100m_ft_fs_pu_1v2  "IO8_FT 100MHz fast speed @ 1.2V pullup"
io8_100m_ft_fs_pd_1v2  "IO8_FT 100MHz fast speed @ 1.2V pulldown"
io8_100m_ft_ms_1v2  "IO8_FT 100MHz med speed @ 1.2V"
io8_100m_ft_ms_pu_1v2  "IO8_FT 100MHz med speed @ 1.2V pullup"
io8_100m_ft_ms_pd_1v2  "IO8_FT 100MHz med speed @ 1.2V pulldown"
io8_100m_ft_ls_1v2  "IO8_FT 100MHz low speed @ 1.2V"
io8_100m_ft_ls_pu_1v2  "IO8_FT 100MHz low speed @ 1.2V pullup"
io8_100m_ft_ls_pd_1v2  "IO8_FT 100MHz low speed @ 1.2V pulldown"
io8_100m_ft_hs_1v8  "IO8_FT 100MHz high speed @ 1.8V"
io8_100m_ft_hs_pu_1v8  "IO8_FT 100MHz high speed @ 1.8V pullup"
io8_100m_ft_hs_pd_1v8  "IO8_FT 100MHz high speed @ 1.8V pulldown"
io8_100m_ft_fs_1v8  "IO8_FT 100MHz fast speed @ 1.8V"
io8_100m_ft_fs_pu_1v8  "IO8_FT 100MHz fast speed @ 1.8V pullup"
io8_100m_ft_fs_pd_1v8  "IO8_FT 100MHz fast speed @ 1.8V pulldown"
io8_100m_ft_ms_1v8  "IO8_FT 100MHz med speed @ 1.8V"
io8_100m_ft_ms_pu_1v8  "IO8_FT 100MHz med speed @ 1.8V pullup"
io8_100m_ft_ms_pd_1v8  "IO8_FT 100MHz med speed @ 1.8V pulldown"
io8_100m_ft_ls_1v8  "IO8_FT 100MHz low speed @ 1.8V"
io8_100m_ft_ls_pu_1v8  "IO8_FT 100MHz low speed @ 1.8V pullup"
io8_100m_ft_ls_pd_1v8  "IO8_FT 100MHz low speed @ 1.8V pulldown"
io8_100m_ft_hs_3v3  "IO8_FT 100MHz high speed @ 3.3V"
io8_100m_ft_hs_pu_3v3  "IO8_FT 100MHz high speed @ 3.3V pullup"
io8_100m_ft_hs_pd_3v3  "IO8_FT 100MHz high speed @ 3.3V pulldown"
io8_100m_ft_fs_3v3  "IO8_FT 100MHz fast speed @ 3.3V"
io8_100m_ft_fs_pu_3v3  "IO8_FT 100MHz fast speed @ 3.3V pullup"
io8_100m_ft_fs_pd_3v3  "IO8_FT 100MHz fast speed @ 3.3V pulldown"
io8_100m_ft_ms_3v3  "IO8_FT 100MHz med speed @ 3.3V"
io8_100m_ft_ms_pu_3v3  "IO8_FT 100MHz med speed @ 3.3V pullup"
io8_100m_ft_ms_pd_3v3  "IO8_FT 100MHz med speed @ 3.3V pulldown"
io8_100m_ft_ls_3v3  "IO8_FT 100MHz low speed @ 3.3V"
io8_100m_ft_ls_pu_3v3  "IO8_FT 100MHz low speed @ 3.3V pullup"
io8_100m_ft_ls_pd_3v3  "IO8_FT 100MHz low speed @ 3.3V pulldown"
io8_100m_hslv_ft_hs_1v2  "IO8_FT 100MHz HSLV high speed @ 1.2V"
io8_100m_hslv_ft_hs_pu_1v2  "IO8_FT 100MHz HSLV high speed @ 1.2V pullup"
io8_100m_hslv_ft_hs_pd_1v2  "IO8_FT 100MHz HSLV high speed @ 1.2V pulldown"
io8_100m_hslv_ft_fs_1v2  "IO8_FT 100MHz HSLV fast speed @ 1.2V"
io8_100m_hslv_ft_fs_pu_1v2  "IO8_FT 100MHz HSLV fast speed @ 1.2V pullup"
io8_100m_hslv_ft_fs_pd_1v2  "IO8_FT 100MHz HSLV fast speed @ 1.2V pulldown"
io8_100m_hslv_ft_ms_1v2  "IO8_FT 100MHz HSLV med speed @ 1.2V"
io8_100m_hslv_ft_ms_pu_1v2  "IO8_FT 100MHz HSLV med speed @ 1.2V pullup"
io8_100m_hslv_ft_ms_pd_1v2  "IO8_FT 100MHz HSLV med speed @ 1.2V pulldown"
io8_100m_hslv_ft_ls_1v2  "IO8_FT 100MHz HSLV low speed @ 1.2V"
io8_100m_hslv_ft_ls_pu_1v2  "IO8_FT 100MHz HSLV low speed @ 1.2V pullup"
io8_100m_hslv_ft_ls_pd_1v2  "IO8_FT 100MHz HSLV low speed @ 1.2V pulldown"
io8_100m_hslv_ft_hs_1v8  "IO8_FT 100MHz HSLV high speed @ 1.8V"
io8_100m_hslv_ft_hs_pu_1v8  "IO8_FT 100MHz HSLV high speed @ 1.8V pullup"
io8_100m_hslv_ft_hs_pd_1v8  "IO8_FT 100MHz HSLV high speed @ 1.8V pulldown"
io8_100m_hslv_ft_fs_1v8  "IO8_FT 100MHz HSLV fast speed @ 1.8V"
io8_100m_hslv_ft_fs_pu_1v8  "IO8_FT 100MHz HSLV fast speed @ 1.8V pullup"
io8_100m_hslv_ft_fs_pd_1v8  "IO8_FT 100MHz HSLV fast speed @ 1.8V pulldown"
io8_100m_hslv_ft_ms_1v8  "IO8_FT 100MHz HSLV med speed @ 1.8V"
io8_100m_hslv_ft_ms_pu_1v8  "IO8_FT 100MHz HSLV med speed @ 1.8V pullup"
io8_100m_hslv_ft_ms_pd_1v8  "IO8_FT 100MHz HSLV med speed @ 1.8V pulldown"
io8_100m_hslv_ft_ls_1v8  "IO8_FT 100MHz HSLV low speed @ 1.8V"
io8_100m_hslv_ft_ls_pu_1v8  "IO8_FT 100MHz HSLV low speed @ 1.8V pullup"
io8_100m_hslv_ft_ls_pd_1v8  "IO8_FT 100MHz HSLV low speed @ 1.8V pulldown"
io8_100m_hslv_ft_hs_2v5  "IO8_FT 100MHz HSLV high speed @ 2.5V"
io8_100m_hslv_ft_hs_pu_2v5  "IO8_FT 100MHz HSLV high speed @ 2.5V pullup"
io8_100m_hslv_ft_hs_pd_2v5  "IO8_FT 100MHz HSLV high speed @ 2.5V pulldown"
io8_100m_hslv_ft_fs_2v5  "IO8_FT 100MHz HSLV fast speed @ 2.5V"
io8_100m_hslv_ft_fs_pu_2v5  "IO8_FT 100MHz HSLV fast speed @ 2.5V pullup"
io8_100m_hslv_ft_fs_pd_2v5  "IO8_FT 100MHz HSLV fast speed @ 2.5V pulldown"
io8_100m_hslv_ft_ms_2v5  "IO8_FT 100MHz HSLV med speed @ 2.5V"
io8_100m_hslv_ft_ms_pu_2v5  "IO8_FT 100MHz HSLV med speed @ 2.5V pullup"
io8_100m_hslv_ft_ms_pd_2v5  "IO8_FT 100MHz HSLV med speed @ 2.5V pulldown"
io8_100m_hslv_ft_ls_2v5  "IO8_FT 100MHz HSLV low speed @ 2.5V"
io8_100m_hslv_ft_ls_pu_2v5  "IO8_FT 100MHz HSLV low speed @ 2.5V pullup"
io8_100m_hslv_ft_ls_pd_2v5  "IO8_FT 100MHz HSLV low speed @ 2.5V pulldown"
io8_ft_v33_hs_1v2  "IO8_FT_V33 high speed @ 1.2V"
io8_ft_v33_hs_pu_1v2  "IO8_FT_V33 high speed @ 1.2V pullup"
io8_ft_v33_hs_pd_1v2  "IO8_FT_V33 high speed @ 1.2V pulldown"
io8_ft_v33_fs_1v2  "IO8_FT_V33 fast speed @ 1.2V"
io8_ft_v33_fs_pu_1v2  "IO8_FT_V33 fast speed @ 1.2V pullup"
io8_ft_v33_fs_pd_1v2  "IO8_FT_V33 fast speed @ 1.2V pulldown"
io8_ft_v33_ms_1v2  "IO8_FT_V33 med speed @ 1.2V"
io8_ft_v33_ms_pu_1v2  "IO8_FT_V33 med speed @ 1.2V pullup"
io8_ft_v33_ms_pd_1v2  "IO8_FT_V33 med speed @ 1.2V pulldown"
io8_ft_v33_ls_1v2  "IO8_FT_V33 low speed @ 1.2V"
io8_ft_v33_ls_pu_1v2  "IO8_FT_V33 low speed @ 1.2V pullup"
io8_ft_v33_ls_pd_1v2  "IO8_FT_V33 low speed @ 1.2V pulldown"
io8_ft_v33_hs_1v8  "IO8_FT_V33 high speed @ 1.8V"
io8_ft_v33_hs_pu_1v8  "IO8_FT_V33 high speed @ 1.8V pullup"
io8_ft_v33_hs_pd_1v8  "IO8_FT_V33 high speed @ 1.8V pulldown"
io8_ft_v33_fs_1v8  "IO8_FT_V33 fast speed @ 1.8V"
io8_ft_v33_fs_pu_1v8  "IO8_FT_V33 fast speed @ 1.8V pullup"
io8_ft_v33_fs_pd_1v8  "IO8_FT_V33 fast speed @ 1.8V pulldown"
io8_ft_v33_ms_1v8  "IO8_FT_V33 med speed @ 1.8V"
io8_ft_v33_ms_pu_1v8  "IO8_FT_V33 med speed @ 1.8V pullup"
io8_ft_v33_ms_pd_1v8  "IO8_FT_V33 med speed @ 1.8V pulldown"
io8_ft_v33_ls_1v8  "IO8_FT_V33 low speed @ 1.8V"
io8_ft_v33_ls_pu_1v8  "IO8_FT_V33 low speed @ 1.8V pullup"
io8_ft_v33_ls_pd_1v8  "IO8_FT_V33 low speed @ 1.8V pulldown"
io8_ft_v33_hs_3v3  "IO8_FT_V33 high speed @ 3.3V"
io8_ft_v33_hs_pu_3v3  "IO8_FT_V33 high speed @ 3.3V pullup"
io8_ft_v33_hs_pd_3v3  "IO8_FT_V33 high speed @ 3.3V pulldown"
io8_ft_v33_fs_3v3  "IO8_FT_V33 fast speed @ 3.3V"
io8_ft_v33_fs_pu_3v3  "IO8_FT_V33 fast speed @ 3.3V pullup"
io8_ft_v33_fs_pd_3v3  "IO8_FT_V33 fast speed @ 3.3V pulldown"
io8_ft_v33_ms_3v3  "IO8_FT_V33 med speed @ 3.3V"
io8_ft_v33_ms_pu_3v3  "IO8_FT_V33 med speed @ 3.3V pullup"
io8_ft_v33_ms_pd_3v3  "IO8_FT_V33 med speed @ 3.3V pulldown"
io8_ft_v33_ls_3v3  "IO8_FT_V33 low speed @ 3.3V"
io8_ft_v33_ls_pu_3v3  "IO8_FT_V33 low speed @ 3.3V pullup"
io8_ft_v33_ls_pd_3v3  "IO8_FT_V33 low speed @ 3.3V pulldown"
[Model Selector] io8_100m_usb_id
io8_100m_ft_hs_1v2  "IO8_FT 100MHz high speed @ 1.2V"
io8_100m_ft_hs_pu_1v2  "IO8_FT 100MHz high speed @ 1.2V pullup"
io8_100m_ft_hs_pd_1v2  "IO8_FT 100MHz high speed @ 1.2V pulldown"
io8_100m_ft_fs_1v2  "IO8_FT 100MHz fast speed @ 1.2V"
io8_100m_ft_fs_pu_1v2  "IO8_FT 100MHz fast speed @ 1.2V pullup"
io8_100m_ft_fs_pd_1v2  "IO8_FT 100MHz fast speed @ 1.2V pulldown"
io8_100m_ft_ms_1v2  "IO8_FT 100MHz med speed @ 1.2V"
io8_100m_ft_ms_pu_1v2  "IO8_FT 100MHz med speed @ 1.2V pullup"
io8_100m_ft_ms_pd_1v2  "IO8_FT 100MHz med speed @ 1.2V pulldown"
io8_100m_ft_ls_1v2  "IO8_FT 100MHz low speed @ 1.2V"
io8_100m_ft_ls_pu_1v2  "IO8_FT 100MHz low speed @ 1.2V pullup"
io8_100m_ft_ls_pd_1v2  "IO8_FT 100MHz low speed @ 1.2V pulldown"
io8_100m_ft_hs_1v8  "IO8_FT 100MHz high speed @ 1.8V"
io8_100m_ft_hs_pu_1v8  "IO8_FT 100MHz high speed @ 1.8V pullup"
io8_100m_ft_hs_pd_1v8  "IO8_FT 100MHz high speed @ 1.8V pulldown"
io8_100m_ft_fs_1v8  "IO8_FT 100MHz fast speed @ 1.8V"
io8_100m_ft_fs_pu_1v8  "IO8_FT 100MHz fast speed @ 1.8V pullup"
io8_100m_ft_fs_pd_1v8  "IO8_FT 100MHz fast speed @ 1.8V pulldown"
io8_100m_ft_ms_1v8  "IO8_FT 100MHz med speed @ 1.8V"
io8_100m_ft_ms_pu_1v8  "IO8_FT 100MHz med speed @ 1.8V pullup"
io8_100m_ft_ms_pd_1v8  "IO8_FT 100MHz med speed @ 1.8V pulldown"
io8_100m_ft_ls_1v8  "IO8_FT 100MHz low speed @ 1.8V"
io8_100m_ft_ls_pu_1v8  "IO8_FT 100MHz low speed @ 1.8V pullup"
io8_100m_ft_ls_pd_1v8  "IO8_FT 100MHz low speed @ 1.8V pulldown"
io8_100m_ft_hs_3v3  "IO8_FT 100MHz high speed @ 3.3V"
io8_100m_ft_hs_pu_3v3  "IO8_FT 100MHz high speed @ 3.3V pullup"
io8_100m_ft_hs_pd_3v3  "IO8_FT 100MHz high speed @ 3.3V pulldown"
io8_100m_ft_fs_3v3  "IO8_FT 100MHz fast speed @ 3.3V"
io8_100m_ft_fs_pu_3v3  "IO8_FT 100MHz fast speed @ 3.3V pullup"
io8_100m_ft_fs_pd_3v3  "IO8_FT 100MHz fast speed @ 3.3V pulldown"
io8_100m_ft_ms_3v3  "IO8_FT 100MHz med speed @ 3.3V"
io8_100m_ft_ms_pu_3v3  "IO8_FT 100MHz med speed @ 3.3V pullup"
io8_100m_ft_ms_pd_3v3  "IO8_FT 100MHz med speed @ 3.3V pulldown"
io8_100m_ft_ls_3v3  "IO8_FT 100MHz low speed @ 3.3V"
io8_100m_ft_ls_pu_3v3  "IO8_FT 100MHz low speed @ 3.3V pullup"
io8_100m_ft_ls_pd_3v3  "IO8_FT 100MHz low speed @ 3.3V pulldown"
io8usb_id_nopu  "IOUSB ID @ 3.3V"
io8usb_id_pu  "IOUSB ID @ 3.3V pullup"
[Model Selector] io8_100m_usb_vbus_ft
io8_100m_ft_hs_1v2  "IO8_FT 100MHz high speed @ 1.2V"
io8_100m_ft_hs_pu_1v2  "IO8_FT 100MHz high speed @ 1.2V pullup"
io8_100m_ft_hs_pd_1v2  "IO8_FT 100MHz high speed @ 1.2V pulldown"
io8_100m_ft_fs_1v2  "IO8_FT 100MHz fast speed @ 1.2V"
io8_100m_ft_fs_pu_1v2  "IO8_FT 100MHz fast speed @ 1.2V pullup"
io8_100m_ft_fs_pd_1v2  "IO8_FT 100MHz fast speed @ 1.2V pulldown"
io8_100m_ft_ms_1v2  "IO8_FT 100MHz med speed @ 1.2V"
io8_100m_ft_ms_pu_1v2  "IO8_FT 100MHz med speed @ 1.2V pullup"
io8_100m_ft_ms_pd_1v2  "IO8_FT 100MHz med speed @ 1.2V pulldown"
io8_100m_ft_ls_1v2  "IO8_FT 100MHz low speed @ 1.2V"
io8_100m_ft_ls_pu_1v2  "IO8_FT 100MHz low speed @ 1.2V pullup"
io8_100m_ft_ls_pd_1v2  "IO8_FT 100MHz low speed @ 1.2V pulldown"
io8_100m_ft_hs_1v8  "IO8_FT 100MHz high speed @ 1.8V"
io8_100m_ft_hs_pu_1v8  "IO8_FT 100MHz high speed @ 1.8V pullup"
io8_100m_ft_hs_pd_1v8  "IO8_FT 100MHz high speed @ 1.8V pulldown"
io8_100m_ft_fs_1v8  "IO8_FT 100MHz fast speed @ 1.8V"
io8_100m_ft_fs_pu_1v8  "IO8_FT 100MHz fast speed @ 1.8V pullup"
io8_100m_ft_fs_pd_1v8  "IO8_FT 100MHz fast speed @ 1.8V pulldown"
io8_100m_ft_ms_1v8  "IO8_FT 100MHz med speed @ 1.8V"
io8_100m_ft_ms_pu_1v8  "IO8_FT 100MHz med speed @ 1.8V pullup"
io8_100m_ft_ms_pd_1v8  "IO8_FT 100MHz med speed @ 1.8V pulldown"
io8_100m_ft_ls_1v8  "IO8_FT 100MHz low speed @ 1.8V"
io8_100m_ft_ls_pu_1v8  "IO8_FT 100MHz low speed @ 1.8V pullup"
io8_100m_ft_ls_pd_1v8  "IO8_FT 100MHz low speed @ 1.8V pulldown"
io8_100m_ft_hs_3v3  "IO8_FT 100MHz high speed @ 3.3V"
io8_100m_ft_hs_pu_3v3  "IO8_FT 100MHz high speed @ 3.3V pullup"
io8_100m_ft_hs_pd_3v3  "IO8_FT 100MHz high speed @ 3.3V pulldown"
io8_100m_ft_fs_3v3  "IO8_FT 100MHz fast speed @ 3.3V"
io8_100m_ft_fs_pu_3v3  "IO8_FT 100MHz fast speed @ 3.3V pullup"
io8_100m_ft_fs_pd_3v3  "IO8_FT 100MHz fast speed @ 3.3V pulldown"
io8_100m_ft_ms_3v3  "IO8_FT 100MHz med speed @ 3.3V"
io8_100m_ft_ms_pu_3v3  "IO8_FT 100MHz med speed @ 3.3V pullup"
io8_100m_ft_ms_pd_3v3  "IO8_FT 100MHz med speed @ 3.3V pulldown"
io8_100m_ft_ls_3v3  "IO8_FT 100MHz low speed @ 3.3V"
io8_100m_ft_ls_pu_3v3  "IO8_FT 100MHz low speed @ 3.3V pullup"
io8_100m_ft_ls_pd_3v3  "IO8_FT 100MHz low speed @ 3.3V pulldown"
io8usb_adp "IOUSB ADP @ 3.3V"
io8usb_vbus "IOUSB VBUS @ 3.3V"
[Model Selector] io8_usb_ft
io8_100m_ft_hs_1v2  "IO8_FT 100MHz high speed @ 1.2V"
io8_100m_ft_hs_pu_1v2  "IO8_FT 100MHz high speed @ 1.2V pullup"
io8_100m_ft_hs_pd_1v2  "IO8_FT 100MHz high speed @ 1.2V pulldown"
io8_100m_ft_fs_1v2  "IO8_FT 100MHz fast speed @ 1.2V"
io8_100m_ft_fs_pu_1v2  "IO8_FT 100MHz fast speed @ 1.2V pullup"
io8_100m_ft_fs_pd_1v2  "IO8_FT 100MHz fast speed @ 1.2V pulldown"
io8_100m_ft_ms_1v2  "IO8_FT 100MHz med speed @ 1.2V"
io8_100m_ft_ms_pu_1v2  "IO8_FT 100MHz med speed @ 1.2V pullup"
io8_100m_ft_ms_pd_1v2  "IO8_FT 100MHz med speed @ 1.2V pulldown"
io8_100m_ft_ls_1v2  "IO8_FT 100MHz low speed @ 1.2V"
io8_100m_ft_ls_pu_1v2  "IO8_FT 100MHz low speed @ 1.2V pullup"
io8_100m_ft_ls_pd_1v2  "IO8_FT 100MHz low speed @ 1.2V pulldown"
io8_100m_ft_hs_1v8  "IO8_FT 100MHz high speed @ 1.8V"
io8_100m_ft_hs_pu_1v8  "IO8_FT 100MHz high speed @ 1.8V pullup"
io8_100m_ft_hs_pd_1v8  "IO8_FT 100MHz high speed @ 1.8V pulldown"
io8_100m_ft_fs_1v8  "IO8_FT 100MHz fast speed @ 1.8V"
io8_100m_ft_fs_pu_1v8  "IO8_FT 100MHz fast speed @ 1.8V pullup"
io8_100m_ft_fs_pd_1v8  "IO8_FT 100MHz fast speed @ 1.8V pulldown"
io8_100m_ft_ms_1v8  "IO8_FT 100MHz med speed @ 1.8V"
io8_100m_ft_ms_pu_1v8  "IO8_FT 100MHz med speed @ 1.8V pullup"
io8_100m_ft_ms_pd_1v8  "IO8_FT 100MHz med speed @ 1.8V pulldown"
io8_100m_ft_ls_1v8  "IO8_FT 100MHz low speed @ 1.8V"
io8_100m_ft_ls_pu_1v8  "IO8_FT 100MHz low speed @ 1.8V pullup"
io8_100m_ft_ls_pd_1v8  "IO8_FT 100MHz low speed @ 1.8V pulldown"
io8_100m_ft_hs_3v3  "IO8_FT 100MHz high speed @ 3.3V"
io8_100m_ft_hs_pu_3v3  "IO8_FT 100MHz high speed @ 3.3V pullup"
io8_100m_ft_hs_pd_3v3  "IO8_FT 100MHz high speed @ 3.3V pulldown"
io8_100m_ft_fs_3v3  "IO8_FT 100MHz fast speed @ 3.3V"
io8_100m_ft_fs_pu_3v3  "IO8_FT 100MHz fast speed @ 3.3V pullup"
io8_100m_ft_fs_pd_3v3  "IO8_FT 100MHz fast speed @ 3.3V pulldown"
io8_100m_ft_ms_3v3  "IO8_FT 100MHz med speed @ 3.3V"
io8_100m_ft_ms_pu_3v3  "IO8_FT 100MHz med speed @ 3.3V pullup"
io8_100m_ft_ms_pd_3v3  "IO8_FT 100MHz med speed @ 3.3V pulldown"
io8_100m_ft_ls_3v3  "IO8_FT 100MHz low speed @ 3.3V"
io8_100m_ft_ls_pu_3v3  "IO8_FT 100MHz low speed @ 3.3V pullup"
io8_100m_ft_ls_pd_3v3  "IO8_FT 100MHz low speed @ 3.3V pulldown"
io8_usb_fs_3v3  "IOUSB fast speed @ 3.3V"
io8_usb_fs_pu1_3v3  "IO8USB fast speed @ 3.3V pullup1"
io8_usb_fs_pd1_3v3  "IOUSB fast speed @ 3.3V pulldown1"
io8_usb_ls_3v3  "IOUSB low speed @ 3.3V"
io8_usb_ls_pu1_3v3  "IOUSB low speed @ 3.3V pullup1"
io8_usb_ls_pd1_3v3  "IOUSB low speed @ 3.3V pulldown1"
io8_usb_fs_pu2_3v3  "IOUSB fast speed @ 3.3V pullup2"
io8_usb_fs_pd2_3v3  "IOUSB fast speed @ 3.3V pulldown2"
io8_usb_ls_pu2_3v3  "IOUSB low speed @ 3.3V pullup2"
io8_usb_ls_pd2_3v3  "IOUSB low speed @ 3.3V pulldown2"
[Model Selector] io8_100m_i2c_ft
io8_100m_ft_hs_1v2  "IO8_FT 100MHz high speed @ 1.2V"
io8_100m_ft_hs_pu_1v2  "IO8_FT 100MHz high speed @ 1.2V pullup"
io8_100m_ft_hs_pd_1v2  "IO8_FT 100MHz high speed @ 1.2V pulldown"
io8_100m_ft_fs_1v2  "IO8_FT 100MHz fast speed @ 1.2V"
io8_100m_ft_fs_pu_1v2  "IO8_FT 100MHz fast speed @ 1.2V pullup"
io8_100m_ft_fs_pd_1v2  "IO8_FT 100MHz fast speed @ 1.2V pulldown"
io8_100m_ft_ms_1v2  "IO8_FT 100MHz med speed @ 1.2V"
io8_100m_ft_ms_pu_1v2  "IO8_FT 100MHz med speed @ 1.2V pullup"
io8_100m_ft_ms_pd_1v2  "IO8_FT 100MHz med speed @ 1.2V pulldown"
io8_100m_ft_ls_1v2  "IO8_FT 100MHz low speed @ 1.2V"
io8_100m_ft_ls_pu_1v2  "IO8_FT 100MHz low speed @ 1.2V pullup"
io8_100m_ft_ls_pd_1v2  "IO8_FT 100MHz low speed @ 1.2V pulldown"
io8_100m_ft_hs_1v8  "IO8_FT 100MHz high speed @ 1.8V"
io8_100m_ft_hs_pu_1v8  "IO8_FT 100MHz high speed @ 1.8V pullup"
io8_100m_ft_hs_pd_1v8  "IO8_FT 100MHz high speed @ 1.8V pulldown"
io8_100m_ft_fs_1v8  "IO8_FT 100MHz fast speed @ 1.8V"
io8_100m_ft_fs_pu_1v8  "IO8_FT 100MHz fast speed @ 1.8V pullup"
io8_100m_ft_fs_pd_1v8  "IO8_FT 100MHz fast speed @ 1.8V pulldown"
io8_100m_ft_ms_1v8  "IO8_FT 100MHz med speed @ 1.8V"
io8_100m_ft_ms_pu_1v8  "IO8_FT 100MHz med speed @ 1.8V pullup"
io8_100m_ft_ms_pd_1v8  "IO8_FT 100MHz med speed @ 1.8V pulldown"
io8_100m_ft_ls_1v8  "IO8_FT 100MHz low speed @ 1.8V"
io8_100m_ft_ls_pu_1v8  "IO8_FT 100MHz low speed @ 1.8V pullup"
io8_100m_ft_ls_pd_1v8  "IO8_FT 100MHz low speed @ 1.8V pulldown"
io8_100m_ft_hs_3v3  "IO8_FT 100MHz high speed @ 3.3V"
io8_100m_ft_hs_pu_3v3  "IO8_FT 100MHz high speed @ 3.3V pullup"
io8_100m_ft_hs_pd_3v3  "IO8_FT 100MHz high speed @ 3.3V pulldown"
io8_100m_ft_fs_3v3  "IO8_FT 100MHz fast speed @ 3.3V"
io8_100m_ft_fs_pu_3v3  "IO8_FT 100MHz fast speed @ 3.3V pullup"
io8_100m_ft_fs_pd_3v3  "IO8_FT 100MHz fast speed @ 3.3V pulldown"
io8_100m_ft_ms_3v3  "IO8_FT 100MHz med speed @ 3.3V"
io8_100m_ft_ms_pu_3v3  "IO8_FT 100MHz med speed @ 3.3V pullup"
io8_100m_ft_ms_pd_3v3  "IO8_FT 100MHz med speed @ 3.3V pulldown"
io8_100m_ft_ls_3v3  "IO8_FT 100MHz low speed @ 3.3V"
io8_100m_ft_ls_pu_3v3  "IO8_FT 100MHz low speed @ 3.3V pullup"
io8_100m_ft_ls_pd_3v3  "IO8_FT 100MHz low speed @ 3.3V pulldown"
io8_100m_i2c_ft_1v2  "IO8_FT 100MHz I2C @ 1.2V"
io8_100m_i2c_ft_pu_1v2  "IO8_FT 100MHz I2C @ 1.2V pullup"
io8_100m_i2c_ft_pd_1v2  "IO8_FT 100MHz I2C @ 1.2V pulldown"
io8_100m_i2c_ft_1v8  "IO8_FT 100MHz I2C @ 1.8V"
io8_100m_i2c_ft_pu_1v8  "IO8_FT 100MHz I2C @ 1.8V pullup"
io8_100m_i2c_ft_pd_1v8  "IO8_FT 100MHz I2C @ 1,8V pulldown"
io8_100m_i2c_ft_3v3  "IO8_FT 100MHz I2C @ 3.3V"
io8_100m_i2c_ft_pu_3v3  "IO8_FT 100MHz I2C HSLV @ 3.3V pullup"
io8_100m_i2c_ft_pd_3v3  "IO8_FT 100MHz I2C @ 3.3V pulldown"
[Model Selector] io8_166m_hslv_i2c_ft
io8_166m_ft_hs_1v2  "IO8_FT 166MHz high speed @ 1.2V"
io8_166m_ft_hs_pu_1v2  "IO8_FT 166MHz high speed @ 1.2V pullup"
io8_166m_ft_hs_pd_1v2  "IO8_FT 166MHz high speed @ 1.2V pulldown"
io8_166m_ft_fs_1v2  "IO8_FT 166MHz fast speed @ 1.2V"
io8_166m_ft_fs_pu_1v2  "IO8_FT 166MHz fast speed @ 1.2V pullup"
io8_166m_ft_fs_pd_1v2  "IO8_FT 166MHz fast speed @ 1.2V pulldown"
io8_166m_ft_ms_1v2  "IO8_FT 166MHz med speed @ 1.2V"
io8_166m_ft_ms_pu_1v2  "IO8_FT 166MHz med speed @ 1.2V pullup"
io8_166m_ft_ms_pd_1v2  "IO8_FT 166MHz med speed @ 1.2V pulldown"
io8_166m_ft_ls_1v2  "IO8_FT 166MHz low speed @ 1.2V"
io8_166m_ft_ls_pu_1v2  "IO8_FT 166MHz low speed @ 1.2V pullup"
io8_166m_ft_ls_pd_1v2  "IO8_FT 166MHz low speed @ 1.2V pulldown"
io8_166m_ft_hs_1v8  "IO8_FT 166MHz high speed @ 1.8V"
io8_166m_ft_hs_pu_1v8  "IO8_FT 166MHz high speed @ 1.8V pullup"
io8_166m_ft_hs_pd_1v8  "IO8_FT 166MHz high speed @ 1.8V pulldown"
io8_166m_ft_fs_1v8  "IO8_FT 166MHz fast speed @ 1.8V"
io8_166m_ft_fs_pu_1v8  "IO8_FT 166MHz fast speed @ 1.8V pullup"
io8_166m_ft_fs_pd_1v8  "IO8_FT 166MHz fast speed @ 1.8V pulldown"
io8_166m_ft_ms_1v8  "IO8_FT 166MHz med speed @ 1.8V"
io8_166m_ft_ms_pu_1v8  "IO8_FT 166MHz med speed @ 1.8V pullup"
io8_166m_ft_ms_pd_1v8  "IO8_FT 166MHz med speed @ 1.8V pulldown"
io8_166m_ft_ls_1v8  "IO8_FT 166MHz low speed @ 1.8V"
io8_166m_ft_ls_pu_1v8  "IO8_FT 166MHz low speed @ 1.8V pullup"
io8_166m_ft_ls_pd_1v8  "IO8_FT 166MHz low speed @ 1.8V pulldown"
io8_166m_ft_hs_3v3  "IO8_FT 166MHz high speed @ 3.3V"
io8_166m_ft_hs_pu_3v3  "IO8_FT 166MHz high speed @ 3.3V pullup"
io8_166m_ft_hs_pd_3v3  "IO8_FT 166MHz high speed @ 3.3V pulldown"
io8_166m_ft_fs_3v3  "IO8_FT 166MHz fast speed @ 3.3V"
io8_166m_ft_fs_pu_3v3  "IO8_FT 166MHz fast speed @ 3.3V pullup"
io8_166m_ft_fs_pd_3v3  "IO8_FT 166MHz fast speed @ 3.3V pulldown"
io8_166m_ft_ms_3v3  "IO8_FT 166MHz med speed @ 3.3V"
io8_166m_ft_ms_pu_3v3  "IO8_FT 166MHz med speed @ 3.3V pullup"
io8_166m_ft_ms_pd_3v3  "IO8_FT 166MHz med speed @ 3.3V pulldown"
io8_166m_ft_ls_3v3  "IO8_FT 166MHz low speed @ 3.3V"
io8_166m_ft_ls_pu_3v3  "IO8_FT 166MHz low speed @ 3.3V pullup"
io8_166m_ft_ls_pd_3v3  "IO8_FT 166MHz low speed @ 3.3V pulldown"
io8_166m_hslv_ft_hs_1v2  "IO8_FT 166MHz HSLV high speed @ 1.2V"
io8_166m_hslv_ft_hs_pu_1v2  "IO8_FT 166MHz HSLV high speed @ 1.2V pullup"
io8_166m_hslv_ft_hs_pd_1v2  "IO8_FT 166MHz HSLV high speed @ 1.2V pulldown"
io8_166m_hslv_ft_fs_1v2  "IO8_FT 166MHz HSLV fast speed @ 1.2V"
io8_166m_hslv_ft_fs_pu_1v2  "IO8_FT 166MHz HSLV fast speed @ 1.2V pullup"
io8_166m_hslv_ft_fs_pd_1v2  "IO8_FT 166MHz HSLV fast speed @ 1.2V pulldown"
io8_166m_hslv_ft_ms_1v2  "IO8_FT 166MHz HSLV med speed @ 1.2V"
io8_166m_hslv_ft_ms_pu_1v2  "IO8_FT 166MHz HSLV med speed @ 1.2V pullup"
io8_166m_hslv_ft_ms_pd_1v2  "IO8_FT 166MHz HSLV med speed @ 1.2V pulldown"
io8_166m_hslv_ft_ls_1v2  "IO8_FT 166MHz HSLV low speed @ 1.2V"
io8_166m_hslv_ft_ls_pu_1v2  "IO8_FT 166MHz HSLV low speed @ 1.2V pullup"
io8_166m_hslv_ft_ls_pd_1v2  "IO8_FT 166MHz HSLV low speed @ 1.2V pulldown"
io8_166m_hslv_ft_hs_1v8  "IO8_FT 166MHz HSLV high speed @ 1.8V"
io8_166m_hslv_ft_hs_pu_1v8  "IO8_FT 166MHz HSLV high speed @ 1.8V pullup"
io8_166m_hslv_ft_hs_pd_1v8  "IO8_FT 166MHz HSLV high speed @ 1.8V pulldown"
io8_166m_hslv_ft_fs_1v8  "IO8_FT 166MHz HSLV fast speed @ 1.8V"
io8_166m_hslv_ft_fs_pu_1v8  "IO8_FT 166MHz HSLV fast speed @ 1.8V pullup"
io8_166m_hslv_ft_fs_pd_1v8  "IO8_FT 166MHz HSLV fast speed @ 1.8V pulldown"
io8_166m_hslv_ft_ms_1v8  "IO8_FT 166MHz HSLV med speed @ 1.8V"
io8_166m_hslv_ft_ms_pu_1v8  "IO8_FT 166MHz HSLV med speed @ 1.8V pullup"
io8_166m_hslv_ft_ms_pd_1v8  "IO8_FT 166MHz HSLV med speed @ 1.8V pulldown"
io8_166m_hslv_ft_ls_1v8  "IO8_FT 166MHz HSLV low speed @ 1.8V"
io8_166m_hslv_ft_ls_pu_1v8  "IO8_FT 166MHz HSLV low speed @ 1.8V pullup"
io8_166m_hslv_ft_ls_pd_1v8  "IO8_FT 166MHz HSLV low speed @ 1.8V pulldown"
io8_166m_hslv_ft_hs_2v5  "IO8_FT 166MHz HSLV high speed @ 2.5V"
io8_166m_hslv_ft_hs_pu_2v5  "IO8_FT 166MHz HSLV high speed @ 2.5V pullup"
io8_166m_hslv_ft_hs_pd_2v5  "IO8_FT 166MHz HSLV high speed @ 2.5V pulldown"
io8_166m_hslv_ft_fs_2v5  "IO8_FT 166MHz HSLV fast speed @ 2.5V"
io8_166m_hslv_ft_fs_pu_2v5  "IO8_FT 166MHz HSLV fast speed @ 2.5V pullup"
io8_166m_hslv_ft_fs_pd_2v5  "IO8_FT 166MHz HSLV fast speed @ 2.5V pulldown"
io8_166m_hslv_ft_ms_2v5  "IO8_FT 166MHz HSLV med speed @ 2.5V"
io8_166m_hslv_ft_ms_pu_2v5  "IO8_FT 166MHz HSLV med speed @ 2.5V pullup"
io8_166m_hslv_ft_ms_pd_2v5  "IO8_FT 166MHz HSLV med speed @ 2.5V pulldown"
io8_166m_hslv_ft_ls_2v5  "IO8_FT 166MHz HSLV low speed @ 2.5V"
io8_166m_hslv_ft_ls_pu_2v5  "IO8_FT 166MHz HSLV low speed @ 2.5V pullup"
io8_166m_hslv_ft_ls_pd_2v5  "IO8_FT 166MHz HSLV low speed @ 2.5V pulldown"
io8_166m_i2c_ft_1v2  "IO8_FT 166MHz I2C @ 1.2V"
io8_166m_i2c_ft_pu_1v2  "IO8_FT 166MHz I2C @ 1.2V pullup"
io8_166m_i2c_ft_pd_1v2  "IO8_FT 166MHz I2C @ 1.2V pulldown"
io8_166m_i2c_ft_1v8  "IO8_FT 166MHz I2C @ 1.8V"
io8_166m_i2c_ft_pu_1v8  "IO8_FT 166MHz I2C @ 1.8V pullup"
io8_166m_i2c_ft_pd_1v8  "IO8_FT 166MHz I2C @ 1,8V pulldown"
io8_166m_i2c_ft_3v3  "IO8_FT 166MHz I2C @ 3.3V"
io8_166m_i2c_ft_pu_3v3  "IO8_FT 166MHz I2C HSLV @ 3.3V pullup"
io8_166m_i2c_ft_pd_3v3  "IO8_FT 166MHz I2C @ 3.3V pulldown"
| Models and submodels in the file (212): io8_100m_ft_hs_1v2 (I/O), io8_100m_ft_hs_pu_1v2 (I/O), io8_100m_ft_hs_pd_1v2 (I/O), io8_100m_ft_fs_1v2 (I/O), io8_100m_ft_fs_pu_1v2 (I/O), io8_100m_ft_fs_pd_1v2 (I/O), io8_100m_ft_ms_1v2 (I/O), io8_100m_ft_ms_pu_1v2 (I/O), io8_100m_ft_ms_pd_1v2 (I/O), io8_100m_ft_ls_1v2 (I/O), io8_100m_ft_ls_pu_1v2 (I/O), io8_100m_ft_ls_pd_1v2 (I/O), io8_100m_ft_hs_1v8 (I/O), io8_100m_ft_hs_pu_1v8 (I/O), io8_100m_ft_hs_pd_1v8 (I/O), io8_100m_ft_fs_1v8 (I/O), io8_100m_ft_fs_pu_1v8 (I/O), io8_100m_ft_fs_pd_1v8 (I/O), io8_100m_ft_ms_1v8 (I/O), io8_100m_ft_ms_pu_1v8 (I/O), io8_100m_ft_ms_pd_1v8 (I/O), io8_100m_ft_ls_1v8 (I/O), io8_100m_ft_ls_pu_1v8 (I/O), io8_100m_ft_ls_pd_1v8 (I/O), io8_100m_ft_hs_3v3 (I/O), io8_100m_ft_hs_pu_3v3 (I/O), io8_100m_ft_hs_pd_3v3 (I/O), io8_100m_ft_fs_3v3 (I/O), io8_100m_ft_fs_pu_3v3 (I/O), io8_100m_ft_fs_pd_3v3 (I/O), io8_100m_ft_ms_3v3 (I/O), io8_100m_ft_ms_pu_3v3 (I/O), io8_100m_ft_ms_pd_3v3 (I/O), io8_100m_ft_ls_3v3 (I/O), io8_100m_ft_ls_pu_3v3 (I/O), io8_100m_ft_ls_pd_3v3 (I/O), io8_100m_hslv_ft_hs_1v2 (I/O), io8_100m_hslv_ft_hs_pu_1v2 (I/O), io8_100m_hslv_ft_hs_pd_1v2 (I/O), io8_100m_hslv_ft_fs_1v2 (I/O), io8_100m_hslv_ft_fs_pu_1v2 (I/O), io8_100m_hslv_ft_fs_pd_1v2 (I/O), io8_100m_hslv_ft_ms_1v2 (I/O), io8_100m_hslv_ft_ms_pu_1v2 (I/O), io8_100m_hslv_ft_ms_pd_1v2 (I/O), io8_100m_hslv_ft_ls_1v2 (I/O), io8_100m_hslv_ft_ls_pu_1v2 (I/O), io8_100m_hslv_ft_ls_pd_1v2 (I/O), io8_100m_hslv_ft_hs_1v8 (I/O), io8_100m_hslv_ft_hs_pu_1v8 (I/O), io8_100m_hslv_ft_hs_pd_1v8 (I/O), io8_100m_hslv_ft_fs_1v8 (I/O), io8_100m_hslv_ft_fs_pu_1v8 (I/O), io8_100m_hslv_ft_fs_pd_1v8 (I/O), io8_100m_hslv_ft_ms_1v8 (I/O), io8_100m_hslv_ft_ms_pu_1v8 (I/O), io8_100m_hslv_ft_ms_pd_1v8 (I/O), io8_100m_hslv_ft_ls_1v8 (I/O), io8_100m_hslv_ft_ls_pu_1v8 (I/O), io8_100m_hslv_ft_ls_pd_1v8 (I/O), io8_100m_hslv_ft_hs_2v5 (I/O), io8_100m_hslv_ft_hs_pu_2v5 (I/O), io8_100m_hslv_ft_hs_pd_2v5 (I/O), io8_100m_hslv_ft_fs_2v5 (I/O), io8_100m_hslv_ft_fs_pu_2v5 (I/O), io8_100m_hslv_ft_fs_pd_2v5 (I/O), io8_100m_hslv_ft_ms_2v5 (I/O), io8_100m_hslv_ft_ms_pu_2v5 (I/O), io8_100m_hslv_ft_ms_pd_2v5 (I/O), io8_100m_hslv_ft_ls_2v5 (I/O), io8_100m_hslv_ft_ls_pu_2v5 (I/O), io8_100m_hslv_ft_ls_pd_2v5 (I/O), io8_166m_ft_hs_1v2 (I/O), io8_166m_ft_hs_pu_1v2 (I/O), io8_166m_ft_hs_pd_1v2 (I/O), io8_166m_ft_fs_1v2 (I/O), io8_166m_ft_fs_pu_1v2 (I/O), io8_166m_ft_fs_pd_1v2 (I/O), io8_166m_ft_ms_1v2 (I/O), io8_166m_ft_ms_pu_1v2 (I/O)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
